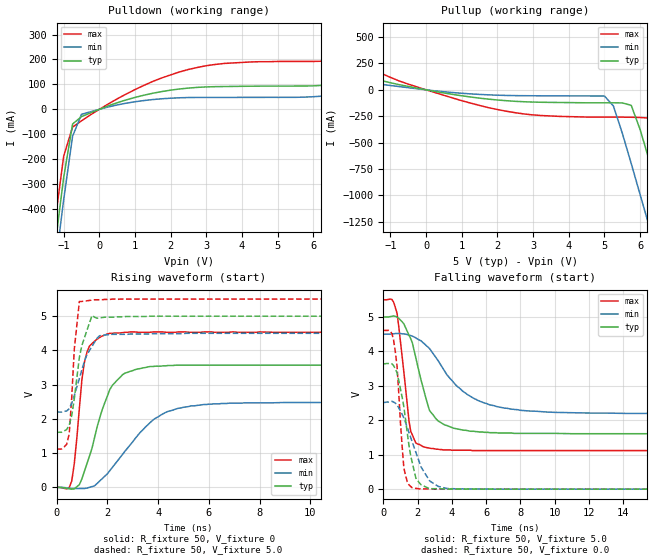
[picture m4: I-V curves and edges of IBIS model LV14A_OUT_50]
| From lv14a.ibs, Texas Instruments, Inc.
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|   Model LV14A_OUT_50
[Model]   LV14A_OUT_50
Model_type  Output
Polarity   Non-Inverting
Vmeas = 2.50v
Cref = 15pf
| variable   typ   min   max
C_comp   4.62pf   3.47pf   5.77pf
[Temperature Range]   25   85   -40
[Voltage Range]   5.0   4.5   5.5
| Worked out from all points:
|   slope of the pulldown table from 0 to 0.75 V, typ, clamps not added: 19.9 ohm
|   slope of the pullup table from 0 to 0.75 V, typ, clamps not added: 17.2 ohm
|   rising waveform, R_fixture 50, V_fixture 0: 20-80 % time 889ps typ, 1.72ns min, 365ps max; typ from 0 V to 3.57 V
|   falling waveform, R_fixture 50, V_fixture 5.0: 20-80 % time 1.06ns typ, 2.44ns min, 573ps max; typ from 5 V to 1.61 V
|   rising waveform, R_fixture 50, V_fixture 5.0: 20-80 % time 440ps typ, 642ps min, 244ps max; typ from 1.61 V to 5 V
|   falling waveform, R_fixture 50, V_fixture 0.0: 20-80 % time 711ps typ, 1.14ns min, 377ps max; typ from 3.64 V to 0 V
[Pulldown]
|   Voltage   I(typ)   I(min)   I(max)
-5V       -5.14A     -5.22A     -5.05A
-1.5V     -853mA     -945mA     -756mA
-1.25V    -557mA     -649mA     -461mA
-1V       -274mA     -363mA     -188mA
-750mV    -58.9mA    -108mA     -71.3mA
-500mV    -29.2mA    -20mA      -46.2mA
0V        -3.33nA    -3.4nA     -3.57nA
1.25V     56.7mA     35.2mA     96mA
2.5V      85.3mA     47.3mA     160mA
3.5V      91.4mA     47.8mA     184mA
6.75V     103mA      58.5mA     199mA
10V       179mA      107mA      329mA
[Pullup]
|   Voltage   I(typ)   I(min)   I(max)
-5V       310mA      167mA      586mA
-3.5V     252mA      143mA      464mA
-750mV    48.6mA     30.8mA     83.5mA
1.5V      -78.8mA    -43.4mA    -148mA
5V        -123mA     -58.9mA    -259mA
5.25V     -123mA     -153mA     -259mA
5.75V     -147mA     -699mA     -260mA
6.25V     -664mA     -1.29A     -268mA
6.5V      -960mA     -1.6A      -403mA
6.75V     -1.26A     -1.9A      -685mA
7.25V     -1.87A     -2.51A     -1.28A
10V       -5.25A     -5.89A     -4.66A
[Ramp]
| variable   typ   min   max
dV/dt_r   2.15E+00/8.67E-10   1.50E+00/1.76E-09   2.72E+00/3.45E-10
dV/dt_f   2.05E+00/1.06E-09   1.39E+00/2.45E-09   2.64E+00/5.67E-10
R_load = 50
[Rising Waveform]
R_fixture = 50
V_fixture = 0
|   Time   V(typ)   V(min)   V(max)
0s        0V         0V         0V
600ps     -51.6mV    -29.5mV    192mV
700ps     -42.5mV    -32.7mV    695mV
1ns       250mV      -32.8mV    3.15V
1.2ns     695mV      -20.7mV    3.95V
2.1ns     2.86V      490mV      4.5V
2.7ns     3.34V      1.06V      4.53V
3.8ns     3.53V      1.97V      4.54V
5.3ns     3.57V      2.38V      4.53V
25ns      3.57V      2.48V      4.53V
[Falling Waveform]
R_fixture = 50
V_fixture = 5.0
V_fixture_min = 4.5
V_fixture_max = 5.5
|   Time   V(typ)   V(min)   V(max)
0s        5V         4.5V       5.5V
500ps     5.02V      4.51V      5.51V
800ps     5V         4.52V      5.11V
1.6ns     4.37V      4.46V      1.68V
2.4ns     2.8V       4.22V      1.22V
2.7ns     2.28V      4.08V      1.19V
3.6ns     1.86V      3.41V      1.14V
4.9ns     1.7V       2.75V      1.13V
7.1ns     1.63V      2.35V      1.12V
25ns      1.61V      2.2V       1.12V
[Rising Waveform]
R_fixture = 50
V_fixture = 5.0
V_fixture_min = 4.5
V_fixture_max = 5.5
|   Time   V(typ)   V(min)   V(max)
0s        1.61V      2.2V       1.12V
400ps     1.69V      2.23V      1.26V
500ps     1.82V      2.3V       1.56V
600ps     2.1V       2.46V      2.64V
700ps     2.59V      2.68V      4.04V
900ps     3.8V       3.18V      5.43V
1.4ns     5.02V      4.12V      5.47V
1.7ns     4.95V      4.43V      5.48V
2ns       4.97V      4.46V      5.49V
25ns      5V         4.5V       5.5V
[Falling Waveform]
R_fixture = 50
V_fixture = 0.0
|   Time   V(typ)   V(min)   V(max)
0s        3.64V      2.52V      4.61V
600ps     3.59V      2.53V      4.33V
800ps     3.38V      2.45V      3.58V
1.2ns     2.39V      2.07V      616mV
1.4ns     1.63V      1.79V      211mV
1.7ns     751mV      1.35V      36.6mV
2ns       247mV      931mV      16mV
2.7ns     13.4mV     244mV      5.29mV
3.7ns     2.87mV     21.6mV     1.44mV
25ns      11.2uV     3.07uV     9.79uV
